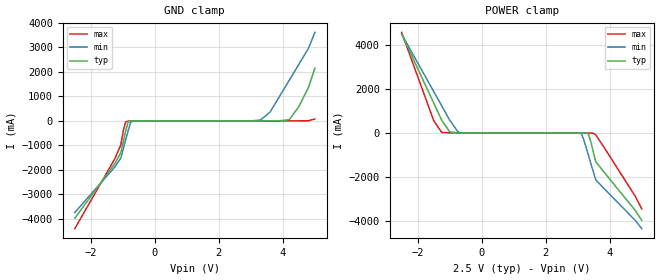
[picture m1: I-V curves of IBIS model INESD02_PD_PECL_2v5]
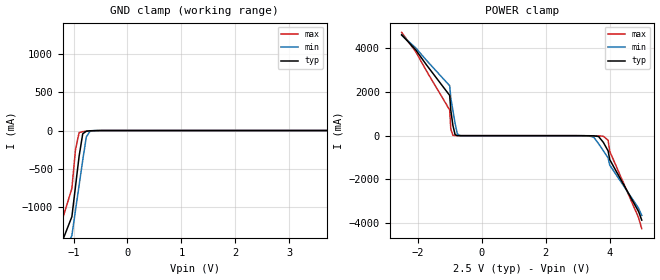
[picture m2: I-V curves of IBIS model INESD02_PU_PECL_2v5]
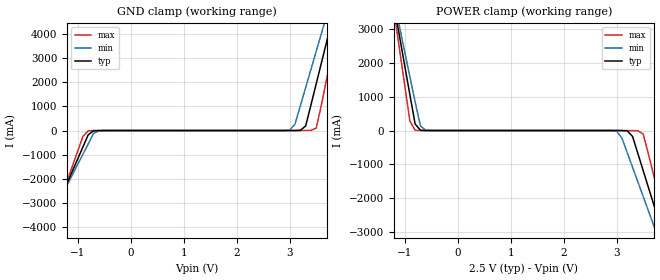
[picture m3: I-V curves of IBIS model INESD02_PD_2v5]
|   This file is an IBIS representation of the   |
|   Integrated Device Technology, Inc.   |
|   ICS87021I   |
|   Div1/Div2 DIFFERENTIAL-TO-LVCMOS/LVTTL CLOCK GENERATOR   |
[IBIS Ver]   4.1
[File name]   87021i.ibs
[File Rev]   1.0
[Date]   16 Jun 2009 | Last modified
|   July 25 2008 | Generated
[Source]   Originated at Integrated Devices Technology, Inc.
[Disclaimer]
IDT hereby grants the user of this IBIS model a non-exclusive,
nontransferable license to use this IBIS model under the following terms.
Before using this IBIS model, the user should read this license.
If the user does not accept these terms,  the IBIS model should be
returned to IDT within 30 days.
   The user is granted this license only to use the IBIS model and
is not granted rights to sell, load, rent, lease or license the IBIS
model in whole or in part, or in modified form to anyone other than
user. User may modify the IBIS model to suit its specific
applications but rights to derivative works and such modifications
shall belong to IDT.
   This IBIS model is provided on an "AS IS" basis and IDT makes
absolutely no warranty with respect to the information contained
herein. IDT DISCLAIMS AND CUSTOMER WAIVES ALL WARRANTIES, EXPRESS
OR IMPLIED, INCLUDING WARRANTIES OF MERCHANTABILITY OR FITNESS FOR
A PARTICULAR PURPOSE. The entire risk as to quality and performance
is with the Customer. ACCORDINGLY, IN NO EVENT SHALL THE COMPANY BE
LIABLE FOR ANY DAMAGES, WHETHER IN CONTRACT OR TORT,INCLUDING ANY
LOST PROFITS OR OTHER INCIDENTAL, CONSEQUENTIAL, EXEMPLARY, OR
PUNITIVE DAMAGES ARISING OUT OF THE USE OR APPLICATION OF THE IBIS
model provided in this package. Further, IDT reserves the right to
make changes without notice to any product herein to improve
reliability, function, or design. IDT does not convey any license
under patent rights or any other intellectual property rights,
including those of third parties.
   IDT is not obligated to provide maintenance or support
for the licensed IBIS model.
[Copyright]   Copyright 2006 by Integrated Device Technology, Inc.
[Component]   ICS87021AMi
[Manufacturer] Integrated Devices Technology, Inc.
[Package]
|SOIC 8 Lead
|   typ   min   max
R_pkg   57.05m   55.5m   58.6m
L_pkg   1.769nH   1.570nH   1.968nH
C_pkg   0.269pF   0.252pF   0.286pF
[Pin] signal_name  model_name   R_pin   L_pin   C_pin
1   CLK   INESD02_PD_PECL   58.6m   1.968n   0.286p
2   nCLK   INESD02_PU_PECL   55.5m   1.570n   0.252p
3   MR   INESD02_PD   55.5m   1.570n   0.252p
4   F_SEL   INESD02_PD   56.6m   1.968n   0.286p
5   GND   GND   58.6m   1.968n   0.286p
6   Q1   COUT05_XFERRES_A   55.5m   1.570n   0.252p
7   Q0   COUT05_XFERRES_A   55.5m   1.570n   0.252p
8   VDD   POWER   56.6m   1.968n   0.286p
[Diff Pin]   inv_pin   vdiff   tdelay_typ  tdelay_min  tdelay_max
  1   2   0.15   0   0   0
[Model Selector] INESD02_PD_PECL
INESD02_PD_PECL_2v5  Buffer selection for 2v5
INESD02_PD_PECL_3v3  Buffer selection for 3v3
[Model Selector] INESD02_PU_PECL
INESD02_PU_PECL_2v5  Buffer selection for 2v5
INESD02_PU_PECL_3v3  Buffer selection for 3v3
[Model Selector] INESD02_PD
INESD02_PD_2v5  Buffer selection for 2v5
INESD02_PD_3v3  Buffer selection for 3v3
[Model Selector] COUT05_XFERRES_A
COUT05_XFERRES_A_2v5  Buffer selection for 2v5
COUT05_XFERRES_A_3v3  Buffer selection for 3v3
| Models and submodels in the file (8): INESD02_PD_PECL_2v5 (Input), INESD02_PU_PECL_2v5 (Input), INESD02_PD_2v5 (Input), COUT05_XFERRES_A_2v5 (Output), INESD02_PD_PECL_3v3 (Input), INESD02_PU_PECL_3v3 (Input), INESD02_PD_3v3 (Input), COUT05_XFERRES_A_3v3 (Output)
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[Model] INESD02_PD_PECL_2v5
Model_type   Input
Polarity   Non-Inverting
Vinl = 0.8V
Vinh = 2.0V
|   typ   min   max
C_comp   2pF   1.5pF   2.5pF
|   typ   min   max
[Voltage range]  2.5V   2.375V   2.625V
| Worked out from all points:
|   GND clamp passes 1 mA (typ) near -0.59 V on its own axis
|   POWER clamp passes 1 mA (typ) near -0.69 V on its own axis
[GND_clamp]
|Voltage   I(typ)   I(min)   I(max)
-2.5V     -3.983A    -3.749A    -4.408A
-1.25V    -1.747A    -1.889A    -1.551A
-1.061V   -1.3A      -1.517A    -979.1mA
-909.1mV  -407.1mA   -774.3mA   -35.24mA
-833.3mV  -48.47mA   -403.4mA   -14.47mA
-757.6mV  -7.272mA   -70.21mA   -9.677mA
-681.8mV  -2.863mA   -7.067mA   -5.73mA
3.3V      167.2uA    32.81mA    49.66uA
3.6V      586.4uA    357.8mA    70.1uA
4.2V      47.81mA    1.661A     649.6uA
4.8V      1.366A     2.965A     5.596mA
5V        2.15A      3.618A     75.79mA
[POWER_clamp]
|Voltage   I(typ)   I(min)   I(max)
-2.5V     4.503A     4.499A     4.579A
-1.5V     1.366A     1.889A     566.5mA
-1.25V    582.4mA    1.237A     24.21mA
-1V       47.81mA    585.7mA    3.595mA
-681.8mV  586.4uA    6.896mA    416.8uA
3.03V     -323.1uA   -3.378mA   -47.98uA
3.106V    -1.127mA   -30.71mA   -286.5uA
3.182V    -2.863mA   -273.7mA   -1.276mA
3.333V    -48.47mA   -1.016A    -7.036mA
3.561V    -1.3A      -2.13A     -81.94mA
4.8V      -3.536A    -3.991A    -2.894A
5V        -3.983A    -4.363A    -3.465A
[Model] INESD02_PU_PECL_2v5
Model_type   Input
Polarity   Non-Inverting
Vinl = .8V
Vinh =  2V
|   typ   min   max
C_comp   2pF   1.5pF   2.5pF
|   typ   min   max
[Voltage range]  2.5V   2.375V   2.625V
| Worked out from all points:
|   GND clamp passes 1 mA (typ) near -0.59 V on its own axis
|   POWER clamp passes 1 mA (typ) near -0.70 V on its own axis
[GND_clamp]
|Voltage   I(typ)   I(min)   I(max)
-2.5V     -3.894A    -3.674A    -4.294A
-1.25V    -1.521A    -1.7A      -1.261A
-1.031V   -1.125A    -1.372A    -755.3mA
-896.9mV  -335.4mA   -714.7mA   -27.06mA
-695.9mV  -3.401mA   -10.7mA    -6.467mA
3.995V    711.6uA    10.32mA    481.3uA
4.062V    4.029mA    88.04mA    1.401mA
4.129V    40.44mA    547.3mA    3.341mA
4.196V    445.8mA    1.124A     14.79mA
4.263V    1.139A     1.7A       275.9mA
4.5V      1.832A     2.277A     1.163A
5V        3.219A     3.431A     2.937A
[POWER_clamp]
|Voltage   I(typ)   I(min)   I(max)
-2.5V     4.617A     4.594A     4.726A
-1V       1.842A     2.286A     1.176A
-963.9mV  1.149A     1.709A     289.6mA
-896.9mV  456.4mA    1.132A     15.33mA
-829.9mV  42.02mA    556.1mA    3.389mA
-762.9mV  4.159mA    91.01mA    1.421mA
-695.9mV  727.9uA    10.67mA    490.4uA
3.35V     -3.204mA   -9.193mA   -6.2mA
3.8V      -305mA     -689.5mA   -24.7mA
3.95V     -699.9mA   -1.018A    -211mA
4V        -1.095A    -1.346A    -716.4mA
5V        -3.863A    -3.649A    -4.255A
[Model] INESD02_PD_2v5
Model_type   Input
Polarity   Non-Inverting
Vinl = 1.4V
Vinh = 1.85V
|   typ   min   max
C_comp   2pF   1.5pF   2.5pF
|   typ   min   max
[Voltage range]  2.5V   2.375V   2.625V
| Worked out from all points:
|   GND clamp passes 1 mA (typ) near -0.55 V on its own axis
|   POWER clamp passes 1 mA (typ) near -0.60 V on its own axis
[GND_clamp]
|Voltage I(typ)   I(min)   I(max)
-2.5V     -8.775A    -7.892A    -10.18A
-1.6V     -4.218A    -4.001A    -4.586A
-900mV    -678.5mA   -979.3mA   -237.6mA
-800mV    -173.9mA   -548.7mA   -10.83mA
-600mV    -1.629mA   -8.74mA    -911.1uA
3V        133.3uA    17.16mA    56.6uA
3.1V      660.9uA    273.5mA    60.87uA
3.3V      191.6mA    1.785A     327.9uA
3.5V      1.949A     3.298A     103.6mA
3.7V      3.723A     4.812A     2.189A
3.9V      5.498A     6.327A     4.369A
5V        15.27A     14.67A     16.38A
[POWER_clamp]
|Voltage   I(typ)   I(min)   I(max)
-2.5V     15.27A     13.72A     17.74A
-1.2V     3.723A     3.866A     3.551A
-1.1V     2.836A     3.109A     2.461A
-900mV    1.063A     1.596A     283.3mA
-800mV    191.6mA    840.1mA    6.189mA
-600mV    660.9uA    8.845mA    114.2uA
3V        -338.1uA   -16.36mA   -12.68uA
3.4V      -678.5mA   -1.518A    -7.183mA
3.5V      -1.183A    -1.95A     -99.52mA
3.7V      -2.195A    -2.813A    -1.324A
4V        -3.712A    -4.109A    -3.188A
5V        -8.775A    -8.432A    -9.404A
